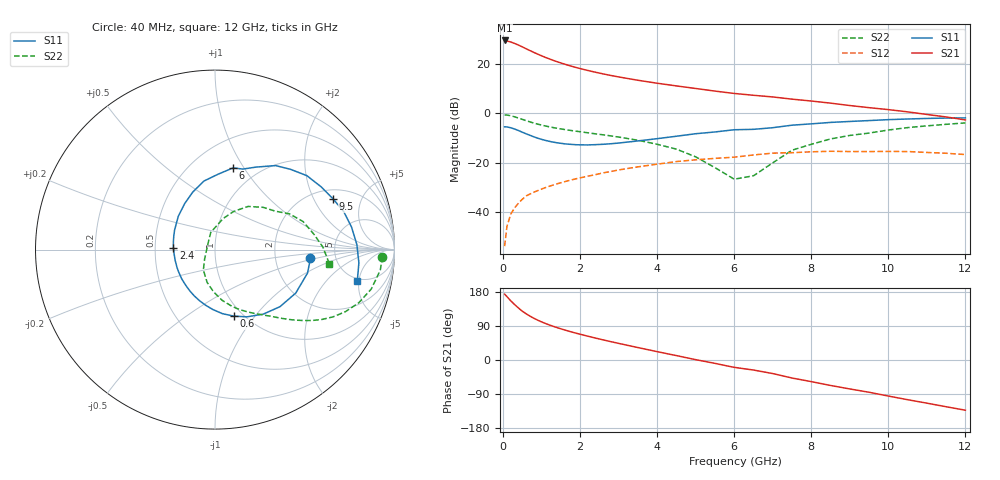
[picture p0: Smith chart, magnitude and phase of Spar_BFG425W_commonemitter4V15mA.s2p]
! Filename: 415bfg425.001
! BFG425W Field C1
! V1=8.370E-001V,V2=4.000E+000V, I1=1.767E-004A, I2=1.500E-002A
# GHz  S  MA  R 50
!  S11  S21  S12  S22
!Freq(GHz)  Mag  Ang  Mag  Ang  Mag  Ang  Mag  Ang
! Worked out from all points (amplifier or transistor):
!   44 points, 40 MHz to 12 GHz, reference 50 ohm
!   highest |S21| = 29.7 dB at 40 MHz (marker M1)
!   |S21| within 3 dB of that: start of sweep to 550.5 MHz
!   unconditionally stable (mu >= 1): start of sweep to 40.81 MHz; 1.594 GHz to end of sweep
!   at 700 MHz: K = 0.67, MSG = 29.2 dB, |S12| = -32.8 dB
!   at 2.4 GHz: K = 1.14, MAG = 18.6 dB, |S12| = -24.9 dB
!   at 12 GHz: K = 1.36, MAG = 3.5 dB, |S12| = -16.7 dB
!   S11 on the Smith chart (normalised r, x): 40 MHz: 3.22, -0.44; 600 MHz: 0.91, -0.79; 2.4 GHz: 0.62, +0.01; 6 GHz: 0.77, +0.90; 9.5 GHz: 2.47, +2.87; 12 GHz: 4.62, -4.76
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0.04  0.534 -5.3  30.48 173.8  0.002 61.5  0.933 -2.4
0.1  0.532 -14.2  29.64 167.3  0.005 71.3  0.928 -7.1
0.2  0.511 -28.3  28.35 156.1  0.009 71.0  0.898 -14.2
0.3  0.482 -41.2  26.51 146.3  0.012 68.5  0.854 -20.3
0.4  0.449 -53.2  24.54 137.1  0.015 65.2  0.805 -25.4
0.5  0.415 -64.5  22.57 128.8  0.018 62.4  0.757 -29.7
0.6  0.385 -74.3  20.65 121.8  0.021 60.6  0.712 -33.1
0.8  0.334 -92.1  17.41 110.1  0.025 57.5  0.637 -38.4
0.9  0.314 -99.7  16.05 105.1  0.027 56.6  0.606 -40.5
1  0.297 -107.1  14.85 100.6  0.029 55.7  0.58 -42.4
1.2  0.271 -120.4  12.86 92.5  0.033 54.4  0.535 -45.8
1.6  0.241 -144.2  10.04 79.2  0.041 52.0  0.471 -51.5
2.2  0.229 -173.7  7.476 62.8  0.053 47.4  0.404 -60.3
2.4  0.232 177.5  6.88 57.9  0.057 45.6  0.385 -63.4
3.5  0.276 137.9  4.729 32.8  0.082 33.1  0.285 -82.1
4.5  0.344 111.1  3.629 11.6  0.105 19.2  0.188 -103.5
6  0.466 77.6  2.549 -19.4  0.129 -4.8  0.046 157.6
6.5  0.475 70.8  2.341 -26.5  0.143 -7.6  0.054 134.6
8.5  0.657 38.8  1.62 -67.2  0.17 -44.6  0.303 52.5
9.5  0.716 23.3  1.311 -85.1  0.168 -61.5  0.399 32.4
10.5  0.771 9.4  1.077 -104.7  0.168 -80.2  0.515 17.7
12  0.812 -12.5  0.738 -132.5  0.146 -110.6  0.642 -7.0
